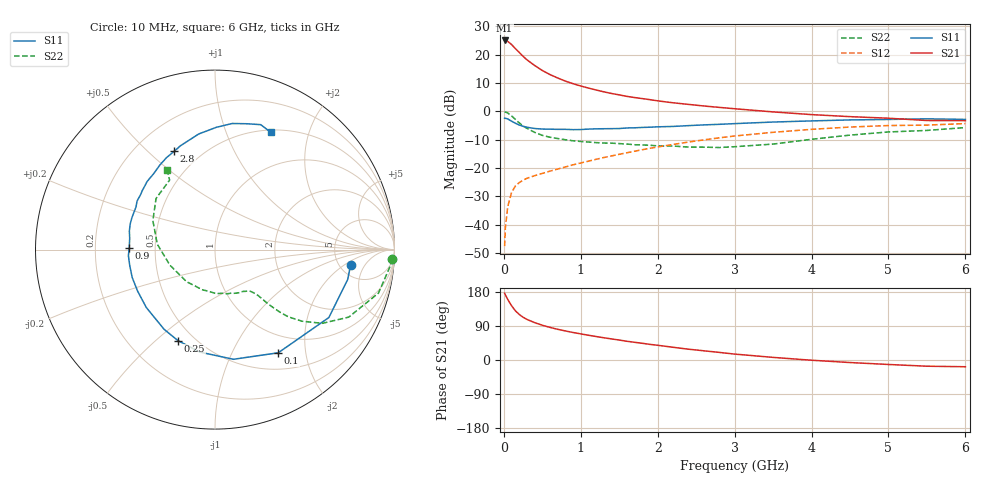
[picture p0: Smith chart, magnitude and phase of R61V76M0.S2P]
! SIEMENS Small Signal Semiconductors
! BFR193
! Si NPN RF Bipolar Junction Transistor in SOT23
! VCE = 1.75 V  IC = 6 mA
! Common Emitter S-Parameters:  May  1996
# GHz  S  MA  R  50
!  f  S11  S21  S12  S22
! GHz  MAG  ANG  MAG  ANG  MAG  ANG  MAG  ANG
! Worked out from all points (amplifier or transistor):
!   36 points, 10 MHz to 6 GHz, reference 50 ohm
!   highest |S21| = 25.1 dB at 10 MHz (marker M1)
!   |S21| within 3 dB of that: start of sweep to 154.9 MHz
!   unconditionally stable (mu >= 1): 841 MHz to 2.014 GHz
!   at 250 MHz: K = 0.49, MSG = 21.9 dB, |S12| = -24.3 dB
!   at 1.4 GHz: K = 1.06, MAG = 9.5 dB, |S12| = -15.7 dB
!   at 6 GHz: K = 0.97, MSG = 0.5 dB, |S12| = -4.3 dB
!   S11 on the Smith chart (normalised r, x): 10 MHz: 6.28, -2.56; 100 MHz: 0.73, -1.53; 250 MHz: 0.41, -0.59; 900 MHz: 0.35, +0.01; 2.8 GHz: 0.36, +0.61; 6 GHz: 0.53, +1.45
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0.01  0.7605 -6.5  17.89 176.2  0.0042 88.5  0.9896 -3.0
0.02  0.7578 -12.7  17.59 171.7  0.0089 84.7  0.9767 -6.1
0.05  0.7388 -30.8  17.23 160.1  0.0207 74.8  0.9425 -14.9
0.1  0.6743 -58.5  15.19 143.3  0.0371 63.6  0.8346 -26.8
0.15  0.6196 -80.5  12.86 129.9  0.0484 56.6  0.7252 -34.5
0.2  0.5772 -98.4  11.04 120.2  0.0556 52.2  0.629 -39.4
0.25  0.5473 -112.2  9.394 112.8  0.0612 49.8  0.5547 -42.5
0.3  0.527 -122.5  8.157 107.2  0.0661 48.8  0.5042 -43.9
0.4  0.5006 -139.9  6.476 98.6  0.0737 48.5  0.4281 -45.6
0.5  0.4893 -151.8  5.283 91.7  0.0807 49.9  0.3786 -46.3
0.6  0.4868 -161.4  4.475 86.0  0.0886 51.5  0.3511 -46.8
0.7  0.4833 -169.2  3.896 81.0  0.0964 52.9  0.333 -47.6
0.9  0.4778 178.6  3.09 72.6  0.1145 55.6  0.3036 -49.8
1.1  0.4884 167.7  2.586 65.3  0.1328 57.4  0.2887 -53.6
1.3  0.4958 159.1  2.22 58.7  0.154 58.1  0.2773 -57.8
1.6  0.5115 148.1  1.845 49.4  0.1868 58.1  0.2659 -66.3
2.2  0.5441 128.8  1.422 33.6  0.2616 54.6  0.2453 -88.3
2.8  0.5929 112.6  1.18 20.1  0.3424 47.6  0.2309 -119.8
3.5  0.6506 98.0  0.982 6.9  0.4287 36.9  0.2657 -160.9
4.5  0.7092 82.2  0.81 -6.7  0.5309 20.7  0.3824 154.9
5.5  0.7413 69.9  0.692 -16.4  0.5748 4.4  0.4626 123.1
6  0.7238 64.6  0.688 -17.8  0.6112 -0.4  0.5199 121.0
